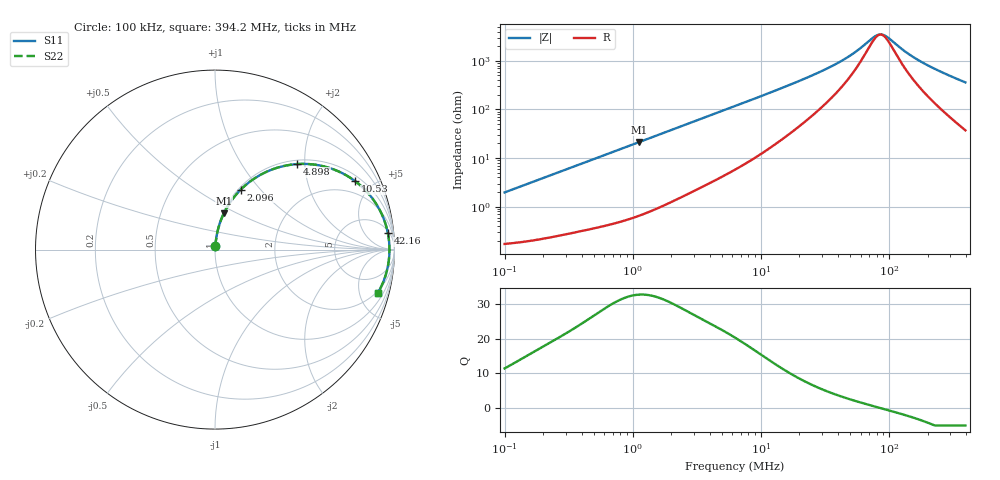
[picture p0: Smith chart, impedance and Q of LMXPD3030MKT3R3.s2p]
! LMXPD3030MKT3R3  S-PARAMETER MODEL  ( General Type )
! Model Generated by TAIYO YUDEN Corporation (http://www.ty-top.com)
! Version 1.0
! TAIYO YUDEN Control No. 191023NI43SB-FBB
! Copyright(c) 2019 TAIYO YUDEN CO.,LTD. All Rights Reserved.
! Product Description (link to TY-COMPAS)
! https://ds.yuden.co.jp/TYCOMPAS/or/detail?pn=LMXPD3030MKT3R3M&u=M
! Products Name : Inductors
! Characteristics :
!  Inductance : 3.3 uH , SRF(min) : 55 MHz , DC Resistance(max) : 0.18 Ohm
!  Rated Current : Saturation :1600 mA , Temp Rise : 1000 mA
!  Case Size : 3.0 x 3.0 / 0.118 x 0.118 [mm/inch] , Thickness : 1.2 / 0.047 [mm/inch]
!  (Conditions: Temperature = 25 degC , DC Bias Current/Voltage = 0A / 0V)
! External Node Assignments :
!  1  o---GGG---o  2
! GND o---------o GND
! Frequency Range : 0.1MHz  -  394.189695MHz  [ 402 STEP ]
# MHz S RI R 50
! Freq[MHz].  S11 Real  S11 Imag  S21 Real  S21 Imag  S12 Real  S12 Imag  S22 Real  S22 Imag
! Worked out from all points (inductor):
!   401 points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, 100 kHz to 394.2 MHz, reference 50 ohm
!   read as one part in series: L = 3.11 uH near 104.2 kHz
!   highest Q = 32.7 at 1.127 MHz (marker M1), where L = 3.03 uH
!   self-resonance near 85.84 MHz
!   S11 on the Smith chart (normalised r, x): 100 kHz: 1.00, +0.04; 2.096 MHz: 1.03, +0.79; 4.898 MHz: 1.08, +1.83; 10.53 MHz: 1.27, +3.94; 42.16 MHz: 7, +19; 394.2 MHz: 1.75, -7.17
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0.1  0.0021 0.0195  0.9979 -0.0195  0.9979 -0.0195  0.0021 0.0195
0.400203  0.009 0.0761  0.991 -0.0761  0.991 -0.0761  0.009 0.0761
0.685491  0.021 0.1277  0.979 -0.1277  0.979 -0.1277  0.021 0.1277
1.126533  0.0496 0.2023  0.9504 -0.2023  0.9504 -0.2023  0.0496 0.2023
1.601627  0.0915 0.2731  0.9085 -0.2731  0.9085 -0.2731  0.0915 0.2731
2.096147  0.1437 0.3345  0.8563 -0.3345  0.8563 -0.3345  0.1437 0.3345
3.106116  0.262 0.4213  0.738 -0.4213  0.738 -0.4213  0.262 0.4213
4.897579  0.4579 0.4766  0.5421 -0.4766  0.5421 -0.4766  0.4579 0.4766
6.278453  0.5752 0.4703  0.4248 -0.4703  0.4248 -0.4703  0.5752 0.4703
10.53378  0.7809 0.3813  0.2191 -0.3813  0.2191 -0.3813  0.7809 0.3813
15.60918  0.8772 0.285  0.1228 -0.285  0.1228 -0.285  0.8772 0.285
25.12657  0.937 0.1793  0.063 -0.1793  0.063 -0.1793  0.937 0.1793
42.15653  0.9632 0.0912  0.0368 -0.0912  0.0368 -0.0912  0.9632 0.0912
54.04257  0.9687 0.057  0.0313 -0.057  0.0313 -0.057  0.9687 0.057
73.71824  0.9718 0.0182  0.0282 -0.0182  0.0282 -0.0182  0.9718 0.0182
80.08146  0.9721 0.00829  0.0279 -0.00829  0.0279 -0.00829  0.9721 0.00829
88.81336  0.9721 -0.00406  0.0279 0.00406  0.0279 0.00406  0.9721 -0.00406
100.5574  0.9718 -0.0189  0.0282 0.0189  0.0282 0.0189  0.9718 -0.0189
134.358  0.9691 -0.0551  0.0309 0.0551  0.0309 0.0551  0.9691 -0.0551
175.8426  0.9634 -0.0922  0.0366 0.0922  0.0366 0.0922  0.9634 -0.0922
260.5674  0.9461 -0.1571  0.0539 0.1571  0.0539 0.1571  0.9461 -0.1571
394.1897  0.9068 -0.2433  0.0932 0.2433  0.0932 0.2433  0.9068 -0.2433
